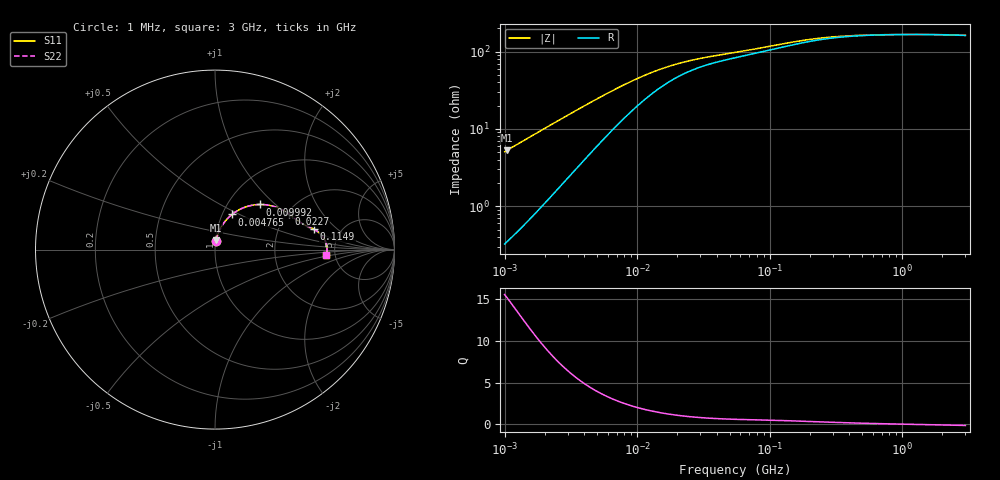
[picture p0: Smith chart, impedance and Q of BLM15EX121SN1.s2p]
! BLM15EX121SN1
# Hz S RI R 50
!Freq.(Hz) S11(Real) S11(Imag) S21(Real) S21(Imag) S12(Real) S12(Imag) S22(Real) S22(Imag)
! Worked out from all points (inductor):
!   401 points, 1 MHz to 3 GHz, reference 50 ohm
!   read as one part in series: L = 805 nH near 1.041 MHz
!   highest Q = 15.2 at 1.041 MHz (marker M1), where L = 806 nH
!   self-resonance near 1.302 GHz
!   S11 on the Smith chart (normalised r, x): 1 MHz: 1.01, +0.10; 4.765 MHz: 1.11, +0.46; 9.992 MHz: 1.39, +0.80; 22.7 MHz: 2.04, +1.04; 114.9 MHz: 3.20, +1.06; 3 GHz: 4.22, -0.39
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1000000  0.00578 0.0502  0.9942 -0.0502  0.9942 -0.0502  0.00578 0.0502
1040844  0.0062 0.0522  0.9938 -0.0522  0.9938 -0.0522  0.0062 0.0522
1553251  0.0128 0.0769  0.9872 -0.0769  0.9872 -0.0769  0.0128 0.0769
2226959  0.0249 0.1074  0.9751 -0.1074  0.9751 -0.1074  0.0249 0.1074
2947212  0.0415 0.1371  0.9585 -0.1371  0.9585 -0.1371  0.0415 0.1371
3823119  0.0656 0.1683  0.9344 -0.1683  0.9344 -0.1683  0.0656 0.1683
4764734  0.0945 0.1956  0.9055 -0.1956  0.9055 -0.1956  0.0945 0.1956
6969505  0.1647 0.2355  0.8353 -0.2355  0.8353 -0.2355  0.1647 0.2355
8345207  0.2055 0.2468  0.7945 -0.2468  0.7945 -0.2468  0.2055 0.2468
9992459  0.2485 0.2513  0.7515 -0.2513  0.7515 -0.2513  0.2485 0.2513
1.196486e7  0.2911 0.2486  0.7089 -0.2486  0.7089 -0.2486  0.2911 0.2486
1.461624e7  0.335 0.2383  0.665 -0.2383  0.665 -0.2383  0.335 0.2383
1.821614e7  0.3766 0.221  0.6234 -0.221  0.6234 -0.221  0.3766 0.221
2.270269e7  0.4101 0.201  0.5899 -0.201  0.5899 -0.201  0.4101 0.201
3.254976e7  0.4505 0.1705  0.5495 -0.1705  0.5495 -0.1705  0.4505 0.1705
5.477226e7  0.4927 0.141  0.5073 -0.141  0.5073 -0.141  0.4927 0.141
1.148668e8  0.5526 0.1132  0.4474 -0.1132  0.4474 -0.1132  0.5526 0.1132
2.094008e8  0.5939 0.0806  0.4061 -0.0806  0.4061 -0.0806  0.5939 0.0806
3.817355e8  0.6151 0.0468  0.3849 -0.0468  0.3849 -0.0468  0.6151 0.0468
8.005644e8  0.6234 0.0159  0.3766 -0.0159  0.3766 -0.0159  0.6234 0.0159
1.613037e9  0.6239 -0.00678  0.3761 0.00678  0.3761 0.00678  0.6239 -0.00678
3e9  0.6192 -0.0286  0.3808 0.0286  0.3808 0.0286  0.6192 -0.0286
